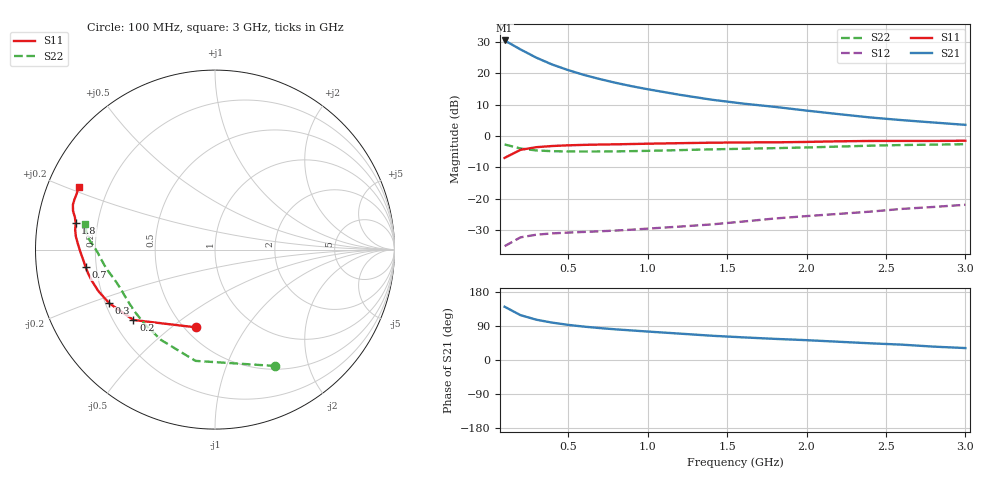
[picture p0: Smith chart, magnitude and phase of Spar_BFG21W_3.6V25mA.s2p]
! Filename: 3_625bfg21.001
! Title: BFG21W
! Bias: Vce=3.6V; Ic=25mA
! Company: NXP Semiconductors NL
! User: Quality&Reliability T&D
! Measure time: 10 Nov 1999 / 11:43:45
#  MHz  S  MA  R 50
! Freq  S11  S21  S12  S22  :
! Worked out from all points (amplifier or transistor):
!   20 points, 100 MHz to 3 GHz, reference 50 ohm
!   highest |S21| = 30.4 dB at 100 MHz (marker M1)
!   |S21| within 3 dB of that: start of sweep to 205.5 MHz
!   unconditionally stable (mu >= 1): 1.128 GHz to end of sweep
!   at 400 MHz: K = 0.48, MSG = 26.9 dB, |S12| = -31.1 dB
!   at 1.2 GHz: K = 1.03, MAG = 19.9 dB, |S12| = -28.9 dB
!   at 3 GHz: K = 1.05, MAG = 11.3 dB, |S12| = -22.0 dB
!   S11 on the Smith chart (normalised r, x): 100 MHz: 0.57, -0.61; 200 MHz: 0.28, -0.35; 300 MHz: 0.22, -0.23; 700 MHz: 0.16, -0.07; 1.8 GHz: 0.12, +0.09; 3 GHz: 0.09, +0.22
100  0.4461 -103.9  33.17 140.6  0.01749 49.5  0.7308 -62.5
200  0.6001 -139.2  23.88 118.3  0.02418 37.0  0.6294 -100.0
300  0.6608 -153.1  17.61 106.3  0.02666 32.1  0.5864 -120.8
400  0.6901 -160.5  13.7 98.5  0.02795 31.0  0.5707 -133.5
500  0.7076 -165.7  11.17 92.7  0.02878 31.2  0.5652 -141.8
600  0.7194 -169.4  9.357 88.1  0.02949 32.7  0.5637 -147.6
700  0.7277 -172.3  8.035 84.2  0.03019 34.8  0.5644 -152.0
800  0.7339 -174.8  7.004 80.9  0.03104 37.3  0.567 -155.6
900  0.7423 -177.1  6.189 78.0  0.03203 40.3  0.5715 -158.6
1000  0.7505 -179.1  5.544 75.1  0.03328 42.9  0.5776 -161.3
1200  0.7657 177.4  4.527 69.7  0.03584 47.9  0.5935 -165.7
1400  0.7785 174.6  3.784 64.1  0.0388 52.4  0.61 -169.2
1600  0.7868 172.0  3.273 59.7  0.04315 56.5  0.6235 -172.2
1800  0.7898 169.3  2.901 55.8  0.04828 60.0  0.6375 -175.4
2000  0.801 167.0  2.53 52.3  0.0527 63.1  0.6542 -178.6
2200  0.8201 164.7  2.226 48.2  0.05712 65.0  0.6754 178.4
2400  0.8302 162.5  1.968 44.1  0.06207 66.0  0.6979 176.1
2600  0.8314 160.4  1.783 40.5  0.06863 66.5  0.7149 174.0
2800  0.8309 157.9  1.634 35.3  0.07376 65.9  0.7256 171.6
3000  0.8375 155.2  1.499 31.5  0.07987 65.9  0.737 168.7
